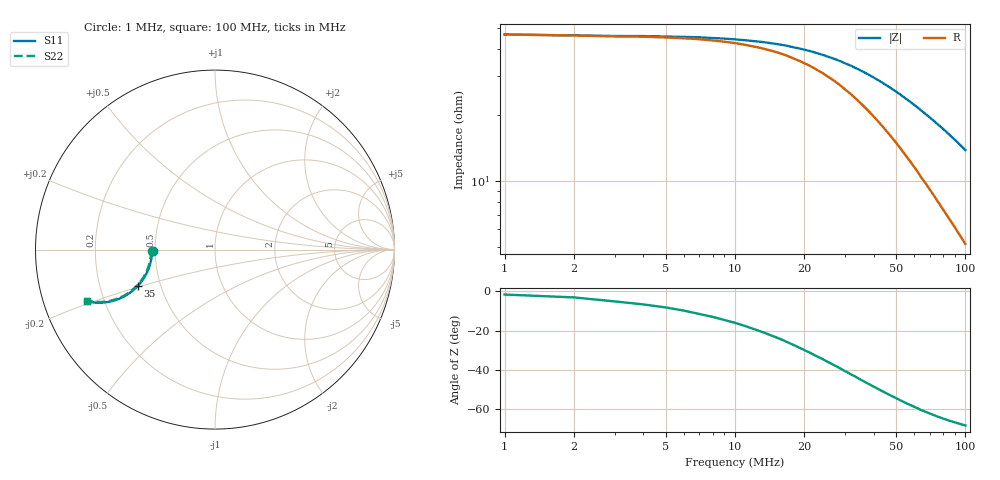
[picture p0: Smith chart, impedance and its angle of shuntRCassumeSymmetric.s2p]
# Hz S RI R 50.0
! written by SimSmith version 18.3b
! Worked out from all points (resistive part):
!   100 points, 1 MHz to 100 MHz, reference 50 ohm
!   read as one part in shunt: R = 46.6 ohm at 1 MHz
!   S11 on the Smith chart (normalised r, x): 1 MHz: 0.49, -0.01; 35 MHz: 0.37, -0.19; 100 MHz: 0.14, -0.19
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1000000  -0.346 -0.00608  0.6512 -0.00685  0.6512 -0.00685  -0.3517 -0.00606
2000000  -0.3492 -0.0118  0.6501 -0.013  0.6501 -0.013  -0.3552 -0.0111
3000000  -0.3515 -0.0206  0.6494 -0.0205  0.6494 -0.0205  -0.357 -0.0201
5000000  -0.3524 -0.0327  0.6484 -0.0331  0.6484 -0.0331  -0.3574 -0.0318
9000000  -0.3558 -0.0585  0.6447 -0.0596  0.6447 -0.0596  -0.3611 -0.0572
1.3e7  -0.3622 -0.0833  0.6386 -0.0848  0.6386 -0.0848  -0.3668 -0.0818
1.8e7  -0.373 -0.1138  0.6276 -0.1154  0.6276 -0.1154  -0.3775 -0.112
2.2e7  -0.3835 -0.1365  0.6175 -0.1388  0.6175 -0.1388  -0.3876 -0.1347
2.7e7  -0.3993 -0.1631  0.6023 -0.166  0.6023 -0.166  -0.4032 -0.1611
3.4e7  -0.4251 -0.1966  0.5767 -0.2  0.5767 -0.2  -0.4287 -0.1946
3.5e7  -0.4291 -0.2012  0.5726 -0.2047  0.5726 -0.2047  -0.4328 -0.1989
4.3e7  -0.4631 -0.2323  0.5395 -0.2371  0.5395 -0.2371  -0.4666 -0.2299
5.1e7  -0.4995 -0.2569  0.5035 -0.2627  0.5035 -0.2627  -0.5029 -0.254
5.6e7  -0.5229 -0.2687  0.4808 -0.2762  0.4808 -0.2762  -0.5264 -0.2659
6.3e7  -0.5558 -0.2815  0.4482 -0.2898  0.4482 -0.2898  -0.5589 -0.2781
6.4e7  -0.5646 -0.2854  0.4456 -0.2929  0.4456 -0.2929  -0.5677 -0.282
6.5e7  -0.5649 -0.2845  0.4387 -0.2933  0.4387 -0.2933  -0.568 -0.2811
6.7e7  -0.5745 -0.2871  0.43 -0.2961  0.43 -0.2961  -0.5775 -0.2835
7.6e7  -0.6151 -0.2946  0.3901 -0.3058  0.3901 -0.3058  -0.6177 -0.2904
8.4e7  -0.6487 -0.2963  0.3569 -0.3094  0.3569 -0.3094  -0.6507 -0.2919
9.1e7  -0.6776 -0.2942  0.3293 -0.3092  0.3293 -0.3092  -0.679 -0.2896
1e8  -0.7107 -0.2888  0.2959 -0.3063  0.2959 -0.3063  -0.7117 -0.284
